|Texas Instruments Incorporated
| Marketing part#   Digital Voltage Range   Package-type   #pins
| DLP9000   3.0V - 3.6V   CLGA   355
[IBIS Ver]   4.1
[File name]   dlp9000.ibs
[File Rev]   1.0
[Date]   10/20/2015
[Source]
| Texas Instruments Incorporated.
| 12500 TI Blvd
| Dallas, TX -75243
[Notes]   Revision History:
| Rev 1.0: 10/20/2015
| - Initial version of the model
| - Model generated from simulations in TISPICE
| - C_comp although listed in numerical order of value are
|   obtained from varying PVT conditions. For PVT conditions for
|   each specific value refer the buffer description under
|   respective [Model]. IBIS model user is responsible for using
|   appropriate C_comp to simulate for Signal Integrity.
| - Warnings regarding combined Non-monotonicity of various models have been
|   reviewd and considered minor and can be ignored.
| - Model names with a trailing _1p8 contain the model for
|   1.8V operation. Model names with a trailing _3p3 contain the model
|   for 3.3V operation.
[Disclaimer]
| This model is designed as an aid for customers of Texas Instruments.
| TI and its licensors and suppliers make no warranties, either expressed
| or implied, with respect to this  model, including the warranties of
| merchantability or fitness for a particular purpose. The model is
| provided solely on an "as is" basis. The entire risk as to its quality
| and performance is with the customer.
[Copyright]
 (C) Copyright 2015 Texas Instruments Incorporated.All rights reserved.
| Component P9_WQXGA_PW 355-pin Device
[Component]   P9_WQXGA_PW
[Manufacturer]   Texas Instruments, Inc.
[Package]
|   typ   min   max
R_pkg   3.65e+00   1.49e+00   8.96e+00
L_pkg   1.56e-08   9.00e-09   4.98e-08
C_pkg   8.06e-12   5.13e-12   1.56e-11
|MBRESET PINS SHOULD BE TIED TO A 250pF CAPACITOR TO GROUND
[Pin]   signal_name   model_name   R_pin   L_pin   C_pin
A1   VSS   GND
A3   VBIAS   POWER
A5   VBIAS   POWER
A7   VBIAS   POWER
A9   VBIAS   POWER
A11   VBIAS   POWER
A13   PG_OFFSET   INPUT   2.56E+00   1.49E-08   6.71E-12
A15   D_CP<2>   LVDS_IN   3.53E+00   1.43E-08   6.31E-12
A17   D_CN<2>   LVDS_IN   3.60E+00   1.44E-08   6.58E-12
A19   A3   INPUT   8.96E+00   4.05E-08   1.53E-11
A21   VCC   POWER
A23   VCC   POWER
A25   VCC   POWER
A27   VCC   POWER
A29   VCC   POWER
B2   VBIAS   POWER
B4   PWRDNZ   INPUT   1.49E+00   9.00E-09   5.13E-12
B6   A2   INPUT   5.77E+00   2.63E-08   1.17E-11
B8   D_AN<11>   LVDS_IN   3.63E+00   1.53E-08   7.24E-12
B10   D_AP<11>   LVDS_IN   3.55E+00   1.54E-08   7.26E-12
B12   VSS   GND
B14   D_AN<13>   LVDS_IN   3.64E+00   1.40E-08   7.00E-12
B16   D_AP<13>   LVDS_IN   3.55E+00   1.43E-08   6.76E-12
B18   VSS   GND
B20   D_CN<4>   LVDS_IN   3.63E+00   1.50E-08   6.76E-12
B22   D_CP<4>   LVDS_IN   3.52E+00   1.39E-08   6.78E-12
B24   VSS   GND
B26   D_CN<8>   LVDS_IN   3.65E+00   1.55E-08   6.15E-12
B28   D_CP<8>   LVDS_IN   3.54E+00   1.43E-08   6.42E-12
B30   VSS   GND
C1   VCC   POWER
C3   IRQZ   OUTPUT   5.16E+00   2.34E-08   1.08E-11
C5   A1   INPUT   5.43E+00   2.47E-08   1.14E-11
C7   VSS   GND
C9   D_AN<9>   LVDS_IN   3.59E+00   1.52E-08   7.57E-12
C11   D_AP<9>   LVDS_IN   3.52E+00   1.51E-08   7.77E-12
C13   VSS   GND
C15   D_CN<0>   LVDS_IN   3.57E+00   1.46E-08   7.18E-12
C17   D_CP<0>   LVDS_IN   3.51E+00   1.40E-08   7.05E-12
C19   VSS   GND
C21   DCLK_CP   LVDS_IN   3.56E+00   1.35E-08   6.55E-12
C23   DCLK_CN   LVDS_IN   3.62E+00   1.54E-08   7.20E-12
C25   VSS   GND
C27   D_CN<10>   LVDS_IN   3.63E+00   1.54E-08   7.00E-12
C29   D_CP<10>   LVDS_IN   3.43E+00   1.45E-08   6.82E-12
C31   VCC   POWER
D2   D_AN<7>   LVDS_IN   3.62E+00   1.50E-08   7.55E-12
D4   D_AP<7>   LVDS_IN   3.43E+00   1.40E-08   7.16E-12
D6   VSS   GND
D8   SCTRL_AN   LVDS_IN   3.66E+00   1.41E-08   7.92E-12
D10   SCTRL_AP   LVDS_IN   3.57E+00   1.51E-08   8.13E-12
D12   VSS   GND
D14   D_AP<15>   LVDS_IN   3.58E+00   1.51E-08   7.68E-12
D16   D_AN<15>   LVDS_IN   3.62E+00   1.43E-08   7.21E-12
D18   VSS   GND
D20   D_CP<6>   LVDS_IN   3.47E+00   1.50E-08   7.78E-12
D22   D_CN<6>   LVDS_IN   3.51E+00   1.40E-08   7.35E-12
D24   VSS   GND
D26   D_CN<12>   LVDS_IN   3.60E+00   1.35E-08   7.62E-12
D28   D_CP<12>   LVDS_IN   3.48E+00   1.36E-08   7.36E-12
D30   VSS   GND
E1   VSS   GND
E3   D_AN<5>   LVDS_IN   3.53E+00   1.45E-08   7.29E-12
E5   D_AP<5>   LVDS_IN   3.49E+00   1.42E-08   7.59E-12
E7   VSS   GND
E9   D_AN<6>   LVDS_IN   3.55E+00   1.40E-08   7.70E-12
E11   D_AP<6>   LVDS_IN   3.54E+00   1.50E-08   7.61E-12
E13   VSS   GND
E15   D_CN<1>   LVDS_IN   3.59E+00   1.51E-08   8.33E-12
E17   D_CP<1>   LVDS_IN   3.54E+00   1.40E-08   8.17E-12
E19   VSS   GND
E21   D_CP<7>   LVDS_IN   3.57E+00   1.45E-08   7.40E-12
E23   D_CN<7>   LVDS_IN   3.63E+00   1.55E-08   7.38E-12
E25   VSS   GND
E27   D_CP<14>   LVDS_IN   3.52E+00   1.42E-08   7.14E-12
E29   D_CN<14>   LVDS_IN   3.59E+00   1.45E-08   7.49E-12
E31   VCC   POWER
F2   D_AP<3>   LVDS_IN   3.46E+00   1.45E-08   7.03E-12
F4   D_AN<3>   LVDS_IN   3.51E+00   1.44E-08   7.23E-12
F6   VSS   GND
F8   D_AP<4>   LVDS_IN   3.57E+00   1.34E-08   7.76E-12
F10   D_AN<4>   LVDS_IN   3.60E+00   1.46E-08   7.84E-12
F12   VSS   GND
F14   D_AN<10>   LVDS_IN   3.56E+00   1.50E-08   8.69E-12
F16   D_AP<10>   LVDS_IN   3.59E+00   1.42E-08   8.45E-12
F18   VSS   GND
F20   D_CN<3>   LVDS_IN   3.43E+00   1.27E-08   8.29E-12
F22   D_CP<3>   LVDS_IN   3.59E+00   1.47E-08   8.55E-12
F24   VSS   GND
F26   D_CP<9>   LVDS_IN   3.58E+00   1.45E-08   7.77E-12
F28   D_CN<9>   LVDS_IN   3.50E+00   1.44E-08   7.46E-12
F30   VSS   GND
G1   MODE1   INPUT   5.18E+00   2.52E-08   1.07E-11
G3   D_AN<1>   LVDS_IN   3.59E+00   1.51E-08   7.47E-12
G5   D_AP<1>   LVDS_IN   3.53E+00   1.43E-08   7.06E-12
G7   VSS   GND
G9   D_AN<2>   LVDS_IN   3.59E+00   1.51E-08   9.32E-12
G11   D_AP<2>   LVDS_IN   3.53E+00   1.37E-08   9.00E-12
G13   VSS   GND
G15   D_AN<12>   LVDS_IN   3.67E+00   1.51E-08   8.97E-12
G17   D_AP<14>   LVDS_IN   3.61E+00   1.48E-08   8.86E-12
G19   VSS   GND
G21   D_CN<5>   LVDS_IN   3.57E+00   1.55E-08   8.87E-12
G23   SCTRL_CN   LVDS_IN   3.54E+00   1.47E-08   8.52E-12
G25   VSS   GND
G27   D_CP<15>   LVDS_IN   3.56E+00   1.41E-08   7.05E-12
G29   D_CN<15>   LVDS_IN   3.58E+00   1.44E-08   7.16E-12
G31   VCC   POWER
H2   DCLK_AN   LVDS_IN   3.67E+00   1.50E-08   7.11E-12
H4   DCLK_AP   LVDS_IN   3.59E+00   1.49E-08   7.03E-12
H6   STROBE   INPUT   4.94E+00   2.38E-08   9.87E-12
H8   D_AP<0>   LVDS_IN   3.53E+00   1.43E-08   9.43E-12
H10   D_AN<0>   LVDS_IN   3.66E+00   1.54E-08   9.74E-12
H12   A0   INPUT   4.74E+00   2.47E-08   1.18E-11
H14   D_AP<12>   LVDS_IN   3.44E+00   1.32E-08   9.27E-12
H16   D_AN<14>   LVDS_IN   3.50E+00   1.27E-08   8.85E-12
H18   VCCI   POWER
H20   D_CP<5>   LVDS_IN   3.38E+00   1.39E-08   8.52E-12
H22   SCTRL_CP   LVDS_IN   3.61E+00   1.44E-08   8.50E-12
H24   VCCI   POWER
H26   D_CN<13>   LVDS_IN   3.45E+00   1.38E-08   7.74E-12
H28   D_CP<13>   LVDS_IN   3.62E+00   1.48E-08   7.44E-12
H30   EN_OFFSET   OUTPUT   7.37E+00   3.72E-08   1.56E-11
J1   MODE0   INPUT   3.90E+00   1.85E-08   8.55E-12
J3   D_AP<8>   LVDS_IN   3.67E+00   1.53E-08   7.56E-12
J5   D_AN<8>   LVDS_IN   3.58E+00   1.47E-08   7.59E-12
J7   N/C   NC
J9   N/C   NC
J11   PROG_FUSE_EN   NC
J13   BIST_B   NC
J15   EN_BIAS   OUTPUT   2.07E+00   1.14E-08   9.43E-12
J17   EN_RESET   OUTPUT   3.47E+00   1.98E-08   1.32E-11
J19   PG_BIAS   INPUT   2.21E+00   1.18E-08   1.10E-11
J21   BIST_D   NC
J23   SINGLE_ASIC_EN   NC
J25   N/C   NC
J27   D_CP<11>   LVDS_IN   3.55E+00   1.44E-08   7.14E-12
J29   D_CN<11>   LVDS_IN   3.57E+00   1.43E-08   7.30E-12
J31   VCC   POWER
K2   VCC   POWER
K4   VSS   GND
K6   VSS   GND
K26   VSS   GND
K28   VSS   GND
K30   VSS   GND
L1   VOFFSET   POWER
L3   MBRST<4>   NC
L5   MBRST<0>   NC
L27   MBRST<13>   NC
L29   MBRST<9>   NC
L31   VRESET   POWER
M2   VSS   GND
M4   MBRST<8>   NC
M6   VCCI   POWER
M26   VCCI   POWER
M28   MBRST<1>   NC
M30   VSS   GND
N1   VOFFSET   POWER
N3   MBRST<12>   NC
N5   VSS   GND
N27   VSS   GND
N29   MBRST<11>   NC
N31   VRESET   POWER
P2   MBRST<6>   NC
P4   MBRST<2>   NC
P6   VCCI   POWER
P26   VCCI   POWER
P28   MBRST<5>   NC
P30   MBRST<3>   NC
R1   VOFFSET   POWER
R3   MBRST<14>   NC
R5   VSS   GND
R27   MBRST<31>   NC
R29   MBRST<17>   NC
R31   VRESET   POWER
T2   VSS   GND
T4   MBRST<10>   NC
T6   VCCI   POWER
T26   VCCI   POWER
T28   MBRST<7>   NC
T30   VSS   GND
U1   VOFFSET   POWER
U3   MBRST<28>   NC
U5   MBRST<24>   NC
U27   VSS   GND
U29   MBRST<25>   NC
U31   VRESET   POWER
V2   VSS   GND
V4   MBRST<16>   NC
V6   VCCI   POWER
V26   VCCI   POWER
V28   MBRST<15>   NC
V30   VSS   GND
W1   VOFFSET   POWER
W3   MBRST<20>   NC
W5   VSS   GND
W27   MBRST<21>   NC
W29   MBRST<23>   NC
W31   VRESET   POWER
Y2   MBRST<26>   NC
Y4   MBRST<18>   NC
Y6   VCCI   POWER
Y26   VCCI   POWER
Y28   VSS   GND
Y30   MBRST<29>   NC
AA1   VOFFSET   POWER
AA3   MBRST<22>   NC
AA5   MBRST<30>   NC
AA27   MBRST<19>   NC
AA29   MBRST<27>   NC
AA31   VRESET   POWER
AB2   VSS   GND
AB4   VSS   GND
AB6   VSS   GND
AB26   VSS   GND
AB28   VSS   GND
AB30   VSS   GND
AC1   VOFFSET   POWER
AC3   SCPDO   OUTPUT   3.36E+00   1.67E-08   8.20E-12
AC5   VSS   GND
AC7   TST_MUX   NC
AC9   TP0   NC
AC11   TP1   NC
AC13   TP2   NC
AC15   BIST_A   NC
AC17   TEMPERATURE   NC
AC19   PG_RESET   INPUT   3.57E+00   1.78E-08   1.19E-11
AC21   BIST_C   NC
AC23   XI2   NC
AC25   XI1   NC
AC27   D_DN<1>   LVDS_IN   3.36E+00   1.40E-08   7.37E-12
AC29   D_DP<1>   LVDS_IN   3.63E+00   1.45E-08   7.09E-12
AC31   VCC   POWER
AD2   SCPDI   INPUT   3.56E+00   1.75E-08   8.23E-12
AD4   SCPENZ   INPUT   3.70E+00   1.74E-08   9.13E-12
AD6   VCCI   POWER
AD8   D_BN<0>   LVDS_IN   3.53E+00   1.45E-08   9.34E-12
AD10   D_BP<0>   LVDS_IN   3.58E+00   1.32E-08   9.26E-12
AD12   VCCI   POWER
AD14   D_BN<13>   LVDS_IN   3.55E+00   1.49E-08   9.22E-12
AD16   D_BN<15>   LVDS_IN   3.67E+00   1.47E-08   8.40E-12
AD18   VCCI   POWER
AD20   D_DP<4>   LVDS_IN   3.09E+00   1.40E-08   8.77E-12
AD22   D_DN<8>   LVDS_IN   3.55E+00   1.27E-08   8.78E-12
AD24   VCCI   POWER
AD26   D_DP<14>   LVDS_IN   3.49E+00   1.41E-08   7.74E-12
AD28   D_DN<14>   LVDS_IN   3.79E+00   1.50E-08   7.62E-12
AD30   VSS   GND
AE1   SCPCLK   INPUT   4.47E+00   2.11E-08   9.04E-12
AE3   D_BN<1>   LVDS_IN   3.44E+00   1.40E-08   7.76E-12
AE5   D_BP<1>   LVDS_IN   3.51E+00   1.41E-08   7.45E-12
AE7   VSS   GND
AE9   D_BP<11>   LVDS_IN   3.47E+00   1.55E-08   9.02E-12
AE11   D_BN<11>   LVDS_IN   3.55E+00   1.40E-08   8.79E-12
AE13   VSS   GND
AE15   D_BP<13>   LVDS_IN   3.16E+00   1.34E-08   9.13E-12
AE17   D_BP<15>   LVDS_IN   3.50E+00   1.44E-08   8.26E-12
AE19   VSS   GND
AE21   D_DN<4>   LVDS_IN   3.51E+00   1.49E-08   8.75E-12
AE23   D_DP<8>   LVDS_IN   3.47E+00   1.40E-08   8.94E-12
AE25   VSS   GND
AE27   D_DP<3>   LVDS_IN   3.60E+00   1.51E-08   7.60E-12
AE29   D_DN<3>   LVDS_IN   3.56E+00   1.49E-08   7.24E-12
AE31   VCC   POWER
AF2   D_BN<3>   LVDS_IN   3.52E+00   1.42E-08   7.26E-12
AF4   D_BP<3>   LVDS_IN   3.60E+00   1.50E-08   6.93E-12
AF6   VSS   GND
AF8   D_BN<2>   LVDS_IN   3.61E+00   1.51E-08   8.67E-12
AF10   D_BP<2>   LVDS_IN   3.50E+00   1.41E-08   9.07E-12
AF12   VSS   GND
AF14   D_BN<10>   LVDS_IN   3.66E+00   1.52E-08   8.66E-12
AF16   D_BP<10>   LVDS_IN   3.53E+00   1.33E-08   8.16E-12
AF18   VSS   GND
AF20   D_DN<5>   LVDS_IN   3.89E+00   1.57E-08   8.99E-12
AF22   D_DP<5>   LVDS_IN   3.62E+00   1.36E-08   8.90E-12
AF24   VSS   GND
AF26   D_DP<12>   LVDS_IN   3.55E+00   1.48E-08   7.49E-12
AF28   D_DN<12>   LVDS_IN   3.48E+00   1.51E-08   7.73E-12
AF30   VSS   GND
AG1   VCC   POWER
AG3   D_BP<4>   LVDS_IN   3.52E+00   1.44E-08   7.10E-12
AG5   D_BN<4>   LVDS_IN   3.54E+00   1.47E-08   7.38E-12
AG7   VSS   GND
AG9   D_BN<6>   LVDS_IN   3.59E+00   1.36E-08   8.47E-12
AG11   D_BP<6>   LVDS_IN   3.47E+00   1.40E-08   8.42E-12
AG13   VSS   GND
AG15   D_BP<14>   LVDS_IN   3.50E+00   1.38E-08   8.00E-12
AG17   D_BN<14>   LVDS_IN   3.65E+00   1.44E-08   7.77E-12
AG19   VSS   GND
AG21   D_DN<9>   LVDS_IN   3.56E+00   1.56E-08   8.13E-12
AG23   D_DP<9>   LVDS_IN   3.27E+00   1.49E-08   7.91E-12
AG25   VSS   GND
AG27   D_DP<7>   LVDS_IN   3.67E+00   1.53E-08   7.64E-12
AG29   D_DN<7>   LVDS_IN   3.55E+00   1.49E-08   7.25E-12
AG31   VCC   POWER
AH2   D_BN<7>   LVDS_IN   3.44E+00   1.49E-08   7.15E-12
AH4   D_BP<7>   LVDS_IN   3.53E+00   1.51E-08   7.08E-12
AH6   VSS   GND
AH8   D_BN<5>   LVDS_IN   3.33E+00   1.37E-08   7.44E-12
AH10   D_BP<5>   LVDS_IN   3.62E+00   1.48E-08   7.38E-12
AH12   VSS   GND
AH14   D_BP<12>   LVDS_IN   3.39E+00   1.43E-08   8.58E-12
AH16   D_BN<12>   LVDS_IN   3.65E+00   1.51E-08   8.39E-12
AH18   VSS   GND
AH20   DCLK_DP   LVDS_IN   3.60E+00   1.44E-08   7.21E-12
AH22   DCLK_DN   LVDS_IN   3.53E+00   1.49E-08   7.26E-12
AH24   VSS   GND
AH26   SCTRL_DP   LVDS_IN   3.29E+00   1.46E-08   7.79E-12
AH28   SCTRL_DN   LVDS_IN   3.29E+00   1.46E-08   7.71E-12
AH30   VSS   GND
AJ1   VSS   GND
AJ3   DCLK_BP   LVDS_IN   3.60E+00   1.53E-08   7.78E-12
AJ5   DCLK_BN   LVDS_IN   3.63E+00   1.49E-08   7.94E-12
AJ7   VSS   GND
AJ9   D_BP<9>   LVDS_IN   3.62E+00   1.41E-08   7.43E-12
AJ11   D_BN<9>   LVDS_IN   3.61E+00   1.40E-08   7.15E-12
AJ13   VSS   GND
AJ15   D_DN<0>   LVDS_IN   3.24E+00   1.38E-08   8.70E-12
AJ17   D_DP<0>   LVDS_IN   3.71E+00   1.50E-08   8.07E-12
AJ19   VSS   GND
AJ21   D_DP<10>   LVDS_IN   3.60E+00   1.47E-08   6.98E-12
AJ23   D_DN<10>   LVDS_IN   3.49E+00   1.40E-08   7.25E-12
AJ25   VSS   GND
AJ27   D_DP<11>   LVDS_IN   3.66E+00   1.56E-08   6.80E-12
AJ29   D_DN<11>   LVDS_IN   3.59E+00   1.51E-08   6.81E-12
AJ31   VCC   POWER
AK2   VCC   POWER
AK4   SEL0   INPUT   1.84E+00   1.30E-08   6.48E-12
AK6   VSS   GND
AK8   SCTRL_BN   LVDS_IN   3.42E+00   1.56E-08   7.32E-12
AK10   SCTRL_BP   LVDS_IN   3.68E+00   1.60E-08   7.14E-12
AK12   VSS   GND
AK14   D_DP<2>   LVDS_IN   3.61E+00   1.51E-08   7.39E-12
AK16   D_DN<2>   LVDS_IN   3.38E+00   1.52E-08   7.43E-12
AK18   VSS   GND
AK20   D_DP<13>   LVDS_IN   3.54E+00   1.45E-08   6.85E-12
AK22   D_DN<13>   LVDS_IN   3.66E+00   1.53E-08   6.64E-12
AK24   OEZ   INPUT   6.33E+00   4.98E-08   1.25E-11
AK26   D_DP<15>   LVDS_IN   3.59E+00   1.45E-08   6.60E-12
AK28   D_DN<15>   LVDS_IN   3.60E+00   1.43E-08   6.57E-12
AK30   VCC   POWER
AL3   VCC   POWER
AL5   VCC   POWER
AL7   VCC   POWER
AL9   D_BN<8>   LVDS_IN   3.56E+00   1.44E-08   6.15E-12
AL11   D_BP<8>   LVDS_IN   3.45E+00   1.45E-08   6.37E-12
AL13   SEL1   INPUT   4.51E+00   2.31E-08   9.55E-12
AL15   D_DN<6>   LVDS_IN   3.25E+00   1.48E-08   6.65E-12
AL17   D_DP<6>   LVDS_IN   3.59E+00   1.50E-08   6.46E-12
AL19   RESETZ   INPUT   4.14E+00   2.11E-08   9.33E-12
AL21   VCC   POWER
AL23   VCC   POWER
AL25   VCC   POWER
AL27   VCC   POWER
AL29   VSS   GND
[Diff Pin]  inv_pin  vdiff  tdelay_typ tdelay_min tdelay_max
A15   A17   200mV   NA   NA   NA
B10   B8   200mV   NA   NA   NA
B16   B14   200mV   NA   NA   NA
B22   B20   200mV   NA   NA   NA
B28   B26   200mV   NA   NA   NA
C11   C9   200mV   NA   NA   NA
C17   C15   200mV   NA   NA   NA
C21   C23   200mV   NA   NA   NA
C29   C27   200mV   NA   NA   NA
D4   D2   200mV   NA   NA   NA
D10  D8   200mV   NA   NA   NA
D14  D16   200mV   NA   NA   NA
D20  D22   200mV   NA   NA   NA
D28   D26   200mV   NA   NA   NA
E5   E3   200mV   NA   NA   NA
E11  E9   200mV   NA   NA   NA
E17   E15   200mV   NA   NA   NA
E21   E23   200mV   NA   NA   NA
E27  E29   200mV   NA   NA   NA
F2   F4   200mV   NA   NA   NA
F8   F10   200mV   NA   NA   NA
F16   F14   200mV   NA   NA   NA
F22  F20   200mV   NA   NA   NA
F26   F28   200mV   NA   NA   NA
G5   G3   200mV   NA   NA   NA
G11   G9   200mV   NA   NA   NA
G17   G15   200mV   NA   NA   NA
H20   G21   200mV   NA   NA   NA
G27  G29   200mV   NA   NA   NA
H4   H2   200mV   NA   NA   NA
H8   H10   200mV   NA   NA   NA
H14   H16   200mV   NA   NA   NA
H22  G23   200mV   NA   NA   NA
H28   H26   200mV   NA   NA   NA
J3   J5   200mV   NA   NA   NA
J27   J29   200mV   NA   NA   NA
AC29   AC27   200mV   NA   NA   NA
AD10   AD8   200mV   NA   NA   NA
AE15   AD14   200mV   NA   NA   NA
AE17   AD16   200mV   NA   NA   NA
AD20   AE21   200mV   NA   NA   NA
AE23   AD22   200mV   NA   NA   NA
AD26   AD28   200mV   NA   NA   NA
AE5   AE3   200mV   NA   NA   NA
AE9   AE11   200mV   NA   NA   NA
AE27   AE29   200mV   NA   NA   NA
AF4   AF2   200mV   NA   NA   NA
AF10   AF8   200mV   NA   NA   NA
AF16   AF14   200mV   NA   NA   NA
AF22   AF20   200mV   NA   NA   NA
AF26   AF28   200mV   NA   NA   NA
AG3   AG5   200mV   NA   NA   NA
AG11  AG9   200mV   NA   NA   NA
AG15  AG17   200mV   NA   NA   NA
AG23   AG21   200mV   NA   NA   NA
AG27   AG29   200mV   NA   NA   NA
AH4   AH2   200mV   NA   NA   NA
AH10   AH8   200mV   NA   NA   NA
AH14   AH16   200mV   NA   NA   NA
AH20   AH22   200mV   NA   NA   NA
AH26   AH28   200mV   NA   NA   NA
AJ3   AJ5   200mV   NA   NA   NA
AJ9   AJ11   200mV   NA   NA   NA
AJ17   AJ15   200mV   NA   NA   NA
AJ21   AJ23   200mV   NA   NA   NA
AJ27   AJ29   200mV   NA   NA   NA
AK10   AK8   200mV   NA   NA   NA
AK14   AK16   200mV   NA   NA   NA
AK20   AK22   200mV   NA   NA   NA
AK26   AK28   200mV   NA   NA   NA
AL11 AL9   200mV   NA   NA   NA
AL17   AL15   200mV   NA   NA   NA
[Series Pin Mapping] pin_2 model_name function_table_group
A15   A17   lvds_term
B10   B8   lvds_term
B16   B14   lvds_term
B22   B20   lvds_term
B28   B26   lvds_term
C11   C9   lvds_term
C17   C15   lvds_term
C21   C23   lvds_term
C29   C27   lvds_term
D4   D2   lvds_term
D10  D8   lvds_term
D14  D16   lvds_term
D20  D22   lvds_term
D28   D26   lvds_term
E5   E3   lvds_term
E11  E9   lvds_term
E17   E15   lvds_term
E21   E23   lvds_term
E27  E29   lvds_term
F2   F4   lvds_term
F8   F10   lvds_term
F16   F14   lvds_term
F22  F20   lvds_term
F26   F28   lvds_term
G5   G3   lvds_term
G11   G9   lvds_term
G17   G15   lvds_term
H20   G21   lvds_term
G27  G29   lvds_term
H4   H2   lvds_term
H8   H10   lvds_term
H14   H16   lvds_term
H22  G23   lvds_term
H28   H26   lvds_term
J3   J5   lvds_term
J27   J29   lvds_term
AC29   AC27   lvds_term
AD10   AD8   lvds_term
AE15   AD14   lvds_term
AE17   AD16   lvds_term
AD20   AE21   lvds_term
AE23   AD22   lvds_term
AD26   AD28   lvds_term
AE5   AE3   lvds_term
AE9   AE11   lvds_term
AE27   AE29   lvds_term
AF4   AF2   lvds_term
AF10   AF8   lvds_term
AF16   AF14   lvds_term
AF22   AF20   lvds_term
AF26   AF28   lvds_term
AG3   AG5   lvds_term
AG11  AG9   lvds_term
AG15  AG17   lvds_term
AG23   AG21   lvds_term
AG27   AG29   lvds_term
AH4   AH2   lvds_term
AH10   AH8   lvds_term
AH14   AH16   lvds_term
AH20   AH22   lvds_term
AH26   AH28   lvds_term
AJ3   AJ5   lvds_term
AJ9   AJ11   lvds_term
AJ17   AJ15   lvds_term
AJ21   AJ23   lvds_term
AJ27   AJ29   lvds_term
AK10   AK8   lvds_term
AK14   AK16   lvds_term
AK20   AK22   lvds_term
AK26   AK28   lvds_term
AL11 AL9   lvds_term
AL17   AL15   lvds_term
|   Model
[Model]   lvds_term
Model_type   Series
C_comp   0  0  0
[Voltage Range]   3.3   3   3.6
[Temperature Range]   25   125   -40
[R series]   100   90   110
| Models and submodels in the file (4): INPUT (Input), LVDS_IN (Input), OUTPUT (Output), lvds_term (Series)
